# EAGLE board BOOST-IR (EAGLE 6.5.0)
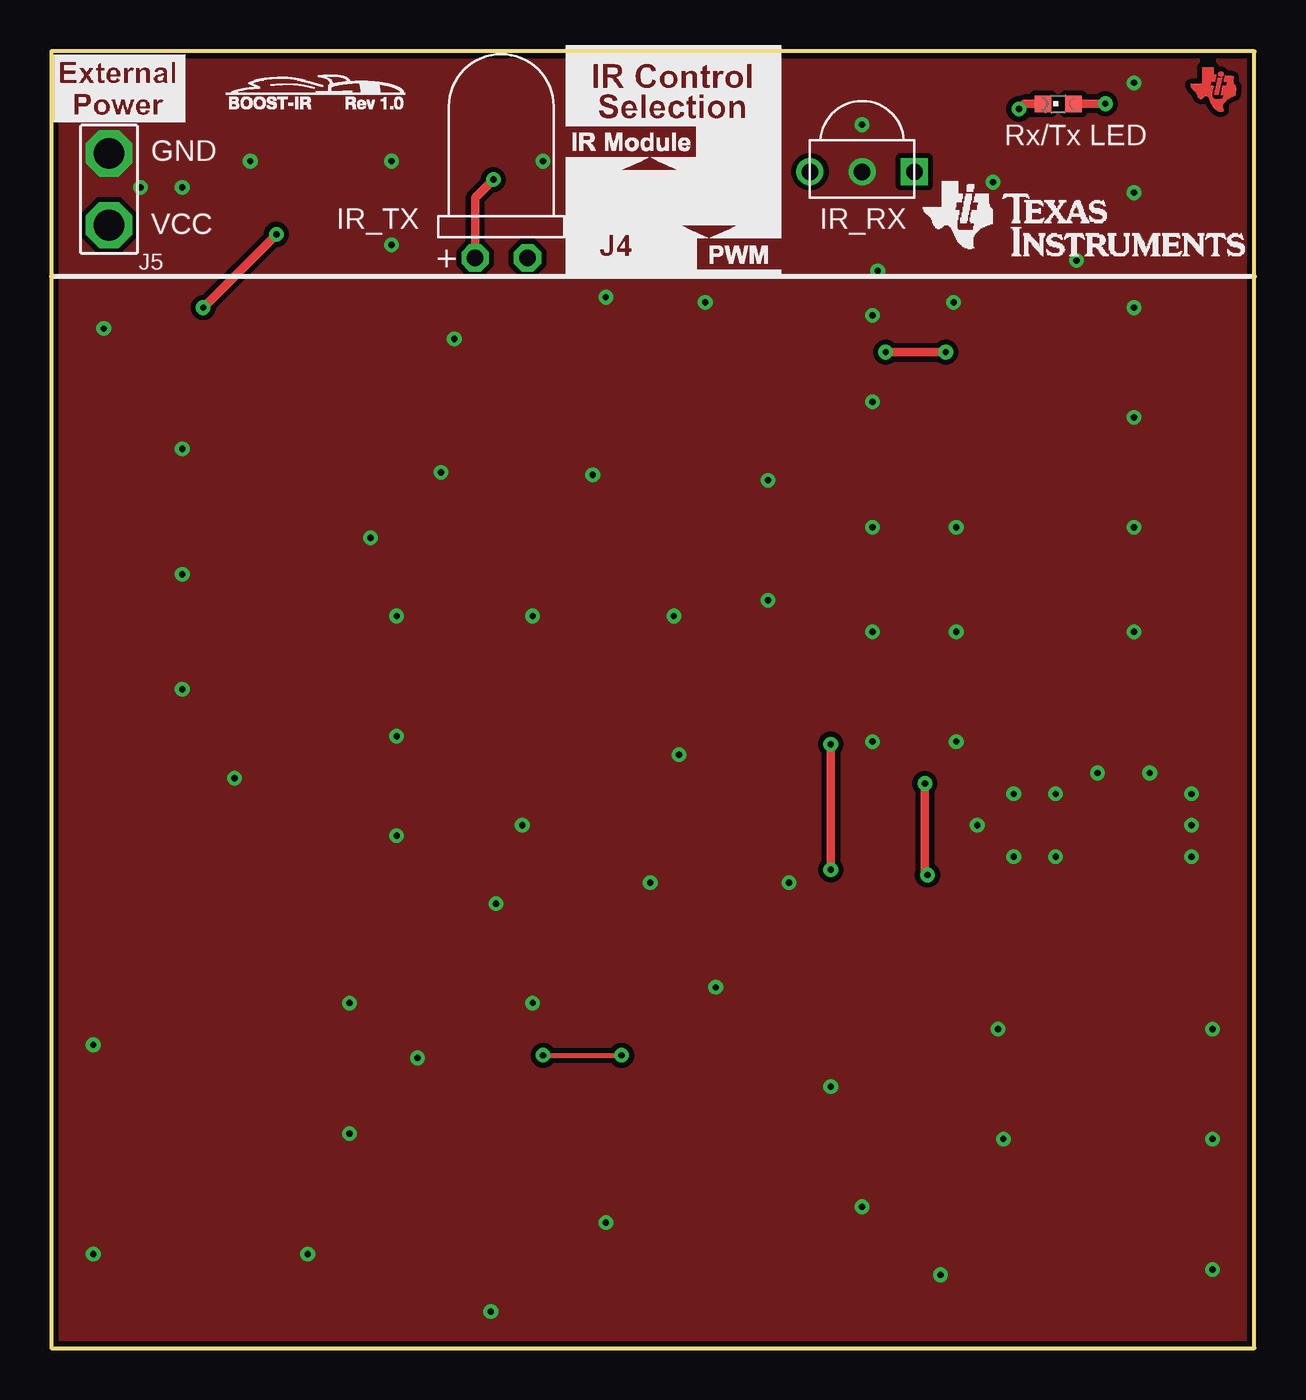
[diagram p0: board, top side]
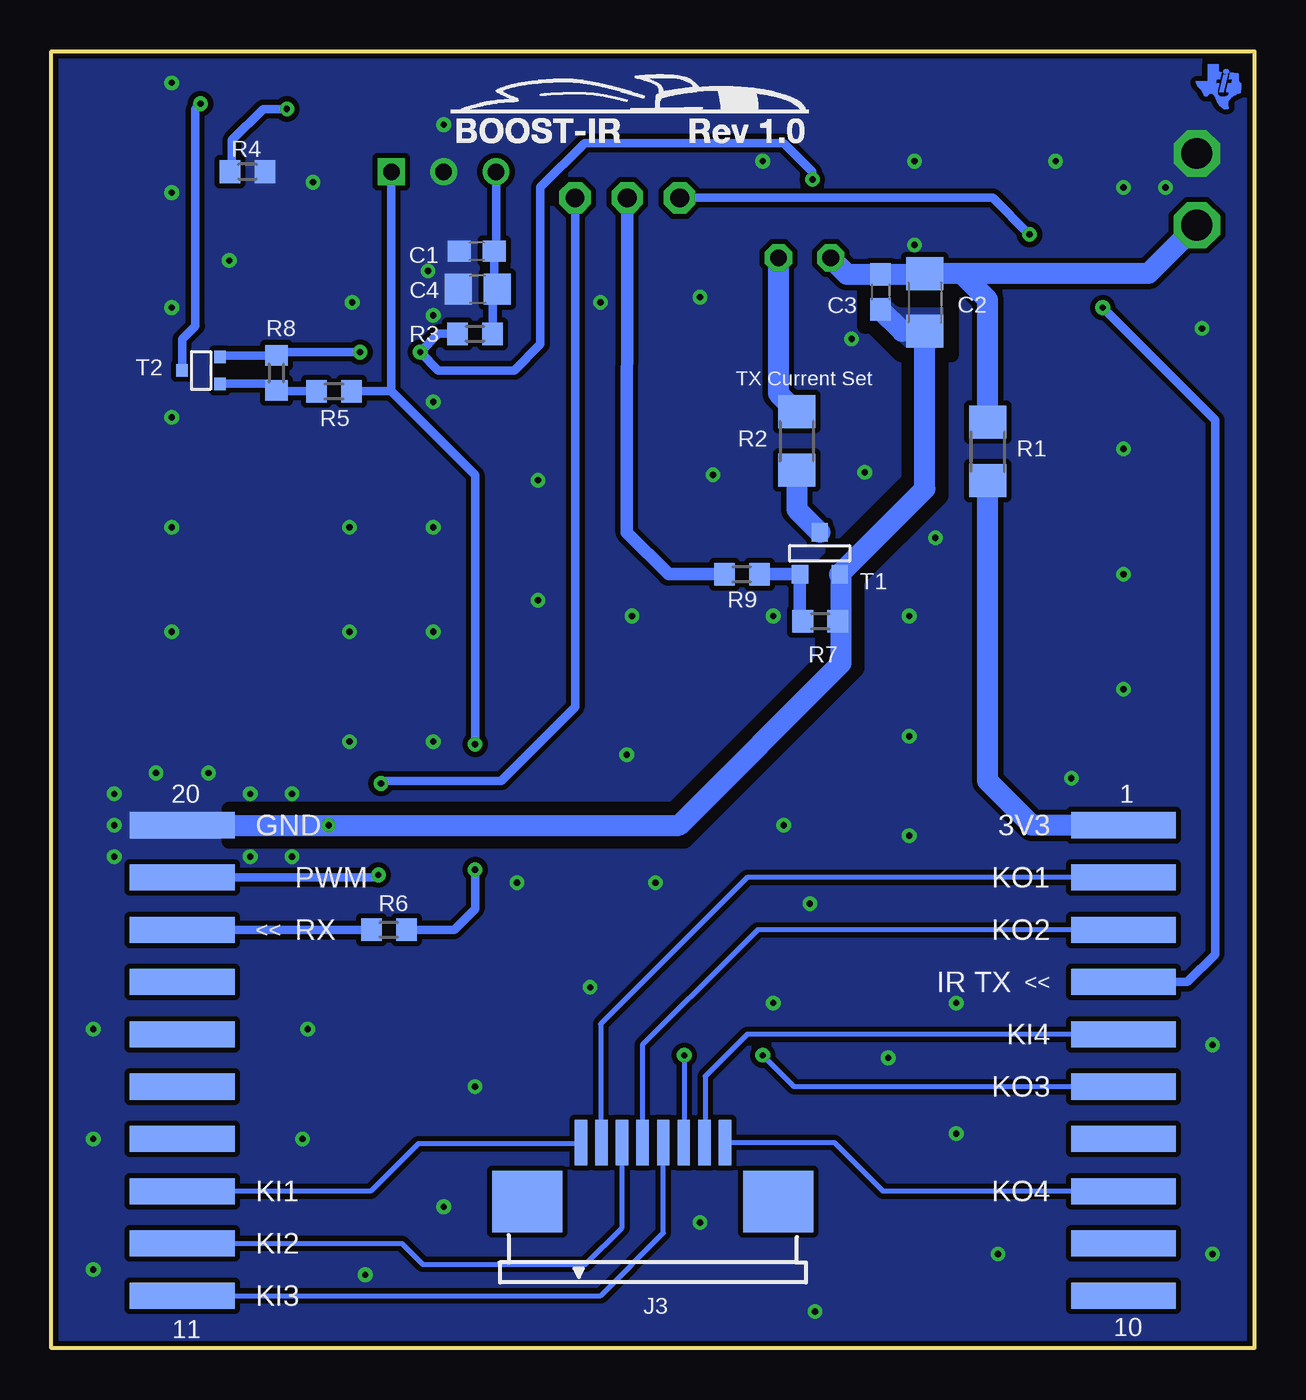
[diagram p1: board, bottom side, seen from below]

Size 58.42 x 62.99 mm. Coordinates in mm from the lower left corner, seen from the top.
Outline: 0,0 58.42,0 58.42,62.99 0,62.99 0,0
Copper layers (1+2*15+16): Top 0.0178mm / dielectric 12mil / Route2 0.0356mm / dielectric 27mil / Route15 0.0356mm / dielectric 12mil / Bottom 0.0178mm
Design rules "MSP430 PCBExpress 4-layer-dietmar": minimum track width 6mil, minimum drill 12mil, track to track 6mil, track to pad 6mil, pad to pad 6mil, via to via 8mil, smd to smd 6mil, copper to edge 8mil, drill to drill 8mil, minimum pad ring 10mil, minimum via ring 8mil, stop-mask expansion 8mil, vias tented up to drill 15mil, thermal gap 8mil
bRestrict: 20 lines

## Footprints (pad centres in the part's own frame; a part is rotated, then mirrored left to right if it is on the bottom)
C0603 = smd 1.1 x 1: 1 -0.85,0; 2 0.85,0
C1206 = smd 1.6 x 1.8: 1 -1.4,0; 2 1.4,0
C0805 = smd 1.3 x 1.5: 1 -0.95,0; 2 0.95,0
TSOP58438 = drill 0.8: GND 0,0; VS 2.54,0 | drill 0.8 square: OUT -2.54,0
IR_LED_PAC = drill 0.813 octagon: A -1.27,0; K 1.27,0
FE10SMD = smd 1.27 x 5.08: 1 0,0; 2 2.54,0; 3 5.08,0; 4 7.62,0; 5 10.16,0; 6 12.7,0; 7 15.24,0; 8 17.78,0; 9 20.32,0; 10 22.86,0
FE10HSMD = smd 1.27 x 5.08: 11 0,0; 12 -2.54,0; 13 -5.08,0; 14 -7.62,0; 15 -10.16,0; 16 -12.7,0; 17 -15.24,0; 18 -17.78,0; 19 -20.32,0; 20 -22.86,0
FPC_IR = smd 0.6 x 2.2: 1 -3.5,4.4; 2 -2.5,4.4; 3 -1.5,4.4; 4 -0.5,4.4; 5 0.5,4.4; 6 1.5,4.4; 7 2.5,4.4; 8 3.5,4.4 | smd 3.4 x 3: P$1 6.096,1.524; P$2 -6.096,1.524
1X03 = drill 0.914 pad 1.524 octagon: 1 -2.54,0; 2 0,0; 3 2.54,0
HEADER1X2 = drill 1.5 pad 2.2 octagon: 1 0,0; 2 3.49,0
CHIPLED_0603 = smd 0.8 x 0.8: A 0,-0.75; C 0,0.75
R1206 = smd 1.6 x 1.803: 1 -1.422,0; 2 1.422,0
R0603 = smd 1 x 1.1: 1 -0.85,0; 2 0.85,0
SOT-23 = smd 0.787 x 0.889: 1 0.025,-1.016; 2 -0.94,1.016; 3 0.991,1.016
SOT323 = smd 0.6 x 0.55: 1 -0.65,-0.825; 2 0.65,-0.825; 3 0,1.025

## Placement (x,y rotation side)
C1  100nF  [C0603]  37.77,53.29 180 bottom
C2  100uF  [C1206]  16,50.8 270 bottom
C3  100nF  [C0603]  18.16,51.31 270 bottom
C4  10uF  [C0805]  37.72,51.44 180 bottom
IR_RX  TSOP58438  [TSOP58438]  39.37,57.15 180 top
IR_TX  TSAL6200  [IR_LED_PAC]  21.84,52.96 0 top
J1  FE10LSMD  [FE10SMD]  6.35,25.4 270 bottom
J2  FE10HSMD  [FE10HSMD]  52.07,2.54 270 bottom
J3  FPC-8-1  [FPC_IR]  29.21,5.59 0 bottom
J4  [1X03]  30.45,55.88 180 top
J5  [HEADER1X2]  2.79,58.04 270 top
LED  BLUE  [CHIPLED_0603]  48.9,60.45 90 top
R1  0  [R1206]  12.95,43.56 90 bottom
R2  47  [R1206]  22.23,44.07 90 bottom
R3  100  [R0603]  37.85,49.28 180 bottom
R4  330  [R0603]  48.9,57.15 180 bottom
R5  10k  [R0603]  44.7,46.48 180 bottom
R6  100  [R0603]  42.04,20.32 180 bottom
R7  100k  [R0603]  21.08,35.31 180 bottom
R8  100k  [R0603]  47.5,47.37 90 bottom
R9  1k  [R0603]  24.89,37.59 0 bottom
T1  FMMT491A  [SOT-23]  21.08,38.61 180 bottom
T2  DMG1013UW  [SOT323]  51.05,47.5 90 bottom
U$1  BOOST-IR_EXTPOWER  [BOOST-IR_EXTPOWER]  0,59.56 0 top
U$2  [TILOGO_SMALL]  56.57,61.42 0 top
U$3  TI_LOGO_LETTERS  [TI_LOGO_WORDS]  41.99,52.3 0 top
U$4  BOOST-IR_LABEL  [BOOST-IR_LABEL]  24.79,52.02 0 top
U$5  BOOST-IR_REV0.1LOGO  [BOOST-IR_LOGO]  21.08,58.55 0 top
U$6  BOOST-IR_REV0.1LOGOSMALL  [BOOST-IR_LOGOSMALL]  8.38,60.2 0 top
U$7  [TILOGO_SMALL]  1.6,61.54 0 bottom

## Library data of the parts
C1-C4 = eagle-ltspice; SPICEMODEL: NONE; SPICEPREFIX: C
IR_RX = TSOP58438; IR: TSOP58438
IR_TX = IrBoosterPack
J1 J2 = LibraryLaunchPad
J3 = FPC_IR
J4 J5 = F5529LP_pinhead
LED = led
R1-R9 = rcl
T1 = zetex; MPN: DSS20201L-7; OC_FARNELL: 1710688; OC_NEWARK: 25R4555
T2 = MSP430G6_LP
U$1 U$3-U$6 = LaunchPad
U$2 U$7 = MSP430_Lab

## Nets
GND: C1.2 C2.2 C3.2 C4.2 IR_RX.GND J2.20 J5.1 R4.1 R7.1 T1.2
IR_MOD: J1.4 J4.3
IR_RX: IR_RX.OUT R5.1 R6.1
IR_TX: J4.2 R9.1
KEYIN1: J2.13 J3.1
KEYIN2: J2.12 J3.3
KEYIN3: J2.11 J3.5
KEYIN4: J1.5 J3.7
KEYOUT1: J1.2 J3.2
KEYOUT2: J1.3 J3.4
KEYOUT3: J1.6 J3.6
KEYOUT4: J1.8 J3.8
N$1: R2.1 T1.1
N$2: IR_TX.K R2.2
N$4: R7.2 R9.2 T1.3
N$5: C1.1 C4.1 IR_RX.VS R3.1
N$9: R5.2 R8.1 T2.1
N$10: LED.A T2.3
N$11: LED.C R4.2
N$12: J2.18 R6.2
N$15: J1.1 R1.1
PWM: J2.19 J4.1
VCC: C2.1 C3.1 IR_TX.A J5.2 R1.2 R3.2 R8.2 T2.2

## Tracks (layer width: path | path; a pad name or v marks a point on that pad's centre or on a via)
GND  (via drill 0.3)
  Bottom 1.016: J2.20 27.94,25.4 20.07,33.27 20.07,37.52 T1.2 16,41.73 C2.2 17.1,49.4 C3.2
  other vias: 6.35,37.59 8.89,27.69 40.13,52.32 39.88,50.16 39.88,45.97 39.88,39.88 39.88,34.8 43.94,39.88 43.94,34.8 43.94,29.46 39.88,29.46 44.96,25.4 46.74,26.92 46.74,23.88 55.37,23.88 55.37,25.4 55.37,26.92 53.34,27.94 50.8,27.94 48.77,26.92 52.58,34.8 52.58,39.88 52.58,45.21 52.58,50.55 52.58,56.13 4.32,56.39 6.35,56.39 9.65,57.66 16.51,57.66 23.88,57.66 39.37,59.44 45.72,56.64 49.78,52.83 43.81,50.8 2.54,49.53 6.35,32 6.35,43.69 2.03,14.73 2.03,4.57 12.45,4.57 26.92,6.1 21.34,1.78 43.18,3.56 39.37,6.86 46.23,10.16 45.97,15.49 37.85,12.7 29.08,22.61 35.81,22.61 32.26,17.53 16.76,24.89 16.76,29.72 16.76,35.56 15.49,39.37 23.37,35.56 30.23,35.56 30.48,28.83 31.75,50.8 26.92,51.05 19.56,49.02 16.51,53.59 52.58,61.47 34.8,42.16 34.8,36.32 26.29,42.42 14.48,16.76 23.37,16.76 21.59,21.59 14.48,10.41 48.77,23.88 56.39,15.49 56.39,10.16 56.39,3.81 22.86,25.4 17.78,14.1 18.92,42.55
  pour Bottom (isolate 0.254, no thermals): 0,62.99 0,0 58.42,0 58.42,62.99
  pour Top (isolate 0.254, no thermals): 0,62.99 0,0 58.42,0 58.42,62.99
IR_MOD  (via drill 0.3)
  Top 0.406: v10.92,54.1 v7.37,50.55
  Bottom 0.406: J1.4 3.25,17.78 1.91,19.13 1.91,45.09 v7.37,50.55 | J4.3 12.7,55.88 v10.92,54.1
IR_RX  (via drill 0.3)
  Top 0.406: v37.85,29.34 v37.85,23.24
  Bottom 0.406: 41.91,46.48 IR_RX.OUT | v37.85,29.34 37.85,42.42 41.91,46.48 | R5.1 41.91,46.48 | v37.85,23.24 37.85,21.34 38.86,20.32 R6.1
IR_TX
  Bottom 0.61: R9.1 28.45,37.59 30.48,39.62 J4.2
KEYIN1
  Bottom 0.254: J2.13 42.93,7.62 40.61,9.93 32.77,9.93 J3.1
KEYIN2
  Bottom 0.254: J2.12 41.4,5.08 40.39,4.06 32.49,4.06 30.71,5.84 | 30.73,5.84 30.71,5.84 | 30.71,5.84 J3.3
KEYIN3
  Bottom 0.254: J2.11 31.75,2.54 28.7,5.59 28.71,5.59 J3.5
KEYIN4
  Bottom 0.254: J1.5 24.64,15.24 26.67,13.21 26.67,11.04 J3.7
KEYOUT1
  Bottom 0.254: J1.2 24.64,22.86 31.75,15.75 31.75,11.04 J3.2
KEYOUT2
  Bottom 0.254: J3.4 29.72,11.01 29.72,14.73 25.15,19.3 24.13,20.32 J1.3
KEYOUT3  (via drill 0.3)
  Top 0.254: v23.88,14.22 v27.69,14.22
  Bottom 0.254: J1.6 22.35,12.7 v23.88,14.22 | v27.69,14.22 27.69,11.03 J3.6
KEYOUT4
  Bottom 0.254: J1.8 18.03,7.62 20.4,9.99 J3.8
N$1
  Bottom 1.016: R2.1 22.23,40.74 T1.1
N$2
  Bottom 1.016: IR_TX.K 23.11,46.38 R2.2
N$4
  Bottom 0.61: R9.2 T1.3 22.07,35.45 R7.2
N$5
  Bottom 0.406: IR_RX.VS 36.83,53.38 C1.1 36.92,51.59 C4.1 37,51.21 R3.1
N$9
  Bottom 0.406: R5.2 47.2,46.48 R8.1 | 47.28,46.48 R8.1 | R8.1 47.83,46.85 T2.1
N$10  (via drill 0.3)
  Top 0.406: v51.18,60.45 LED.A
  Bottom 0.406: T2.3 52.08,49.01 51.44,49.66 51.44,60.2 v51.18,60.45
N$11  (via drill 0.3)
  Top 0.406: LED.C 47.24,60.45 v46.99,60.2
  Bottom 0.406: v46.99,60.2 48.13,60.2 49.66,58.67 49.66,57.24 R4.2
N$12
  Bottom 0.406: J2.18 R6.2
N$15
  Bottom 1.016: J1.1 10.79,25.4 12.95,27.56 R1.1
PWM  (via drill 0.3)
  Top 0.406: v42.42,27.43 42.42,23.11 v42.55,22.99
  Bottom 0.406: J4.1 32.99,31.14 36.58,27.56 42.29,27.56 v42.42,27.43 | v42.55,22.99 42.67,22.86 J2.19
VCC  (via drill 0.3)
  Top 0.406: v40.51,48.39 v43.43,48.39 | IR_TX.A 20.57,55.88 v21.46,56.77
  Bottom 0.406: v21.46,56.77 21.46,57.15 22.86,58.55 32.51,58.55 34.67,56.39 34.67,48.77 35.94,47.5 39.62,47.5 v40.51,48.39 39.62,49.28 R3.2 | v43.43,48.39 47.08,48.39 R8.2 | 47.46,48.44 R8.2 | R8.2 50.23,48.22 T2.2
  Bottom 1.016: J5.2 5.14,52.2 14.22,52.2 | 14.22,52.2 C2.1 16.04,52.16 C3.1 19.77,52.16 IR_TX.A | R1.2 12.95,50.93 14.22,52.2

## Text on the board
tPlace: Rx/Tx LED | GND | VCC | +
bPlace: TX Current Set | 1 | 20 | 3V3 | GND | KO1 | PWM | KO2 | RX | << | << | IR TX | KI4 | KO3 | KO4 | KI1 | KI2 | KI3 | 10 | 11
